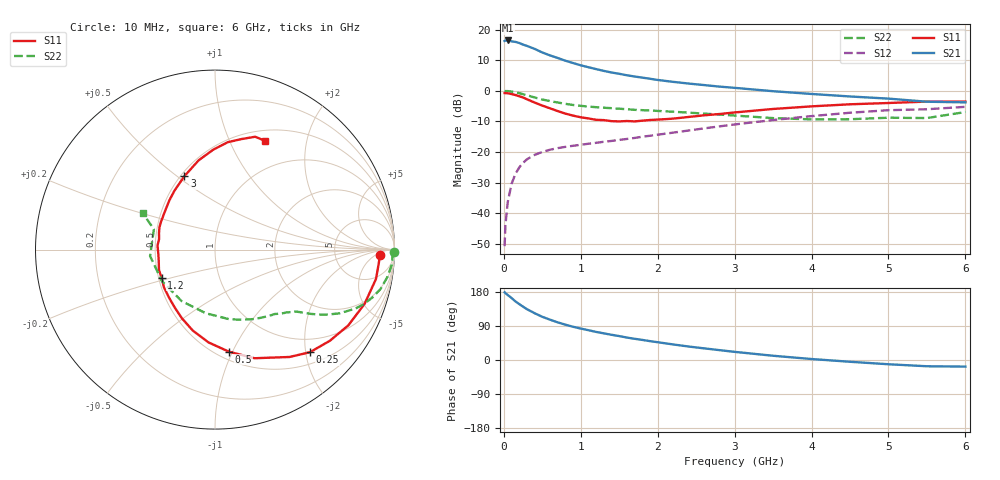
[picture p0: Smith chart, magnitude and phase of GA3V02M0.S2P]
! Infineon Technologies  Discrete & RF Semiconductors
! BF775
! Si NPN RF Bipolar Junction Transistor in SOT23
! VCE = 3 V  IC = 2 mA
! Common Emitter S-Parameters:  May  1996
# GHz  S  MA  R  50
!  f  S11  S21  S12  S22
! GHz  MAG  ANG  MAG  ANG  MAG  ANG  MAG  ANG
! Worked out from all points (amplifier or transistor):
!   36 points, 10 MHz to 6 GHz, reference 50 ohm
!   highest |S21| = 16.5 dB at 50 MHz (marker M1)
!   |S21| within 3 dB of that: start of sweep to 421.6 MHz
!   unconditionally stable (mu >= 1): 1.157 GHz to 3.838 GHz; 5.276 GHz to 5.949 GHz
!   at 250 MHz: K = 0.28, MSG = 19.3 dB, |S12| = -23.5 dB
!   at 1.4 GHz: K = 1.10, MAG = 9.2 dB, |S12| = -16.4 dB
!   at 6 GHz: K = 1.00, MSG = 0.7 dB, |S12| = -5.2 dB
!   S11 on the Smith chart (normalised r, x): 10 MHz: 21, -8; 250 MHz: 0.72, -2.09; 500 MHz: 0.57, -0.97; 1.2 GHz: 0.52, -0.18; 3 GHz: 0.52, +0.53; 6 GHz: 0.63, +1.37
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0.01  0.9192 -1.9  6.532 178.6  0.0029 87.4  0.9972 -0.9
0.02  0.9162 -4.4  6.607 176.5  0.0063 87.6  0.9891 -1.8
0.05  0.9118 -10.3  6.652 171.6  0.015 83.0  0.9899 -4.6
0.1  0.8868 -19.9  6.445 163.7  0.0301 78.0  0.9721 -9.1
0.15  0.8543 -29.6  6.304 154.7  0.0438 72.6  0.948 -13.4
0.2  0.8172 -38.4  6.048 147.6  0.0559 68.1  0.9159 -17.0
0.25  0.7791 -47.2  5.69 140.7  0.0665 63.8  0.8822 -20.2
0.3  0.7285 -55.2  5.418 134.2  0.0761 60.3  0.8483 -22.8
0.4  0.6441 -70.0  4.85 123.5  0.0899 54.3  0.7795 -27.1
0.5  0.5737 -82.3  4.232 114.0  0.1003 50.3  0.7207 -30.2
0.6  0.5179 -94.1  3.793 106.4  0.1091 47.4  0.6805 -32.1
0.8  0.4245 -115.8  3.106 93.2  0.1215 44.2  0.6137 -35.2
0.9  0.3937 -124.6  2.846 87.7  0.1266 43.8  0.587 -36.4
1.1  0.3538 -143.4  2.429 78.6  0.1367 43.4  0.5531 -38.9
1.2  0.3362 -152.4  2.263 74.1  0.1415 43.4  0.5405 -40.2
1.6  0.3212 175.9  1.794 59.2  0.1637 44.8  0.5007 -45.6
2.2  0.3513 142.5  1.402 41.1  0.2076 46.5  0.4557 -56.7
3  0.4433 112.6  1.119 21.5  0.2824 43.5  0.3947 -78.8
3.5  0.5056 100.4  0.986 11.2  0.3334 39.2  0.3584 -98.2
4.5  0.6027 83.2  0.809 -4.7  0.4386 27.1  0.3436 -149.3
5.5  0.6675 70.4  0.664 -16.5  0.5001 11.2  0.359 161.5
6  0.667 65.2  0.648 -17.4  0.5477 6.8  0.4504 153.3
